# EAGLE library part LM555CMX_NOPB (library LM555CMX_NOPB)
Highly stable 555 timer for generating accurate time delays and oscillation Source: Datasheet
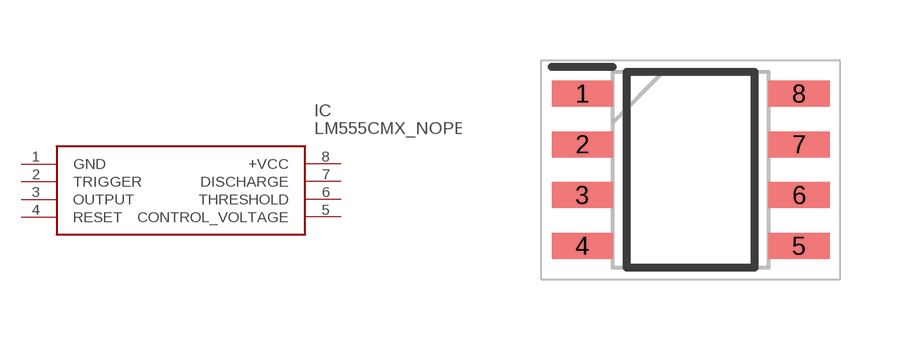
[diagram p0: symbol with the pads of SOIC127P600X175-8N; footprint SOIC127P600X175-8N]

Designator prefix IC

## LM555CMX_NOPB (Arrow_Part_Number: LM555CMX/NOPB; Arrow_Price-Stock: https://www.arrow.com/en/products/lm555cmxnopb/texas-instruments?region=nac; Description: Highly stable 555 timer for generating accurate time delays and oscillation; Height: 1.75mm; Manufacturer_Name: Texas Instruments; Manufacturer_Part_Number: LM555CMX/NOPB; Mouser_Part_Number: 926-LM555CMX/NOPB; Mouser_Price-Stock: https://www.mouser.co.uk/ProductDetail/Texas-Instruments/LM555CMX-NOPB?qs=QbsRYf82W3GHnQuoL%2FmIoA%3D%3D)  [SOIC127P600X175-8N]
1  GND
2  TRIGGER
3  OUTPUT
4  RESET
5  CONTROL_VOLTAGE
6  THRESHOLD
7  DISCHARGE
8  +VCC

## Footprint SOIC127P600X175-8N (pad centres in mm)
D0008A
smd 1.528 x 0.65: 1 -2.711,1.905; 2 -2.711,0.635; 3 -2.711,-0.635; 4 -2.711,-1.905; 5 2.711,-1.905; 6 2.711,-0.635; 7 2.711,0.635; 8 2.711,1.905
